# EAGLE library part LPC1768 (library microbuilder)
LPC1768 100 MHz 32-bit ARM Cortex-M3 based microcontroller featuring a high level of integration and low power consumption. 512 kB Flash, 64 kB SRAM, USB Device/Host/OTG, Ethernet, CAN, I2S, 10-bit DAC Digikey: 568-4796-ND
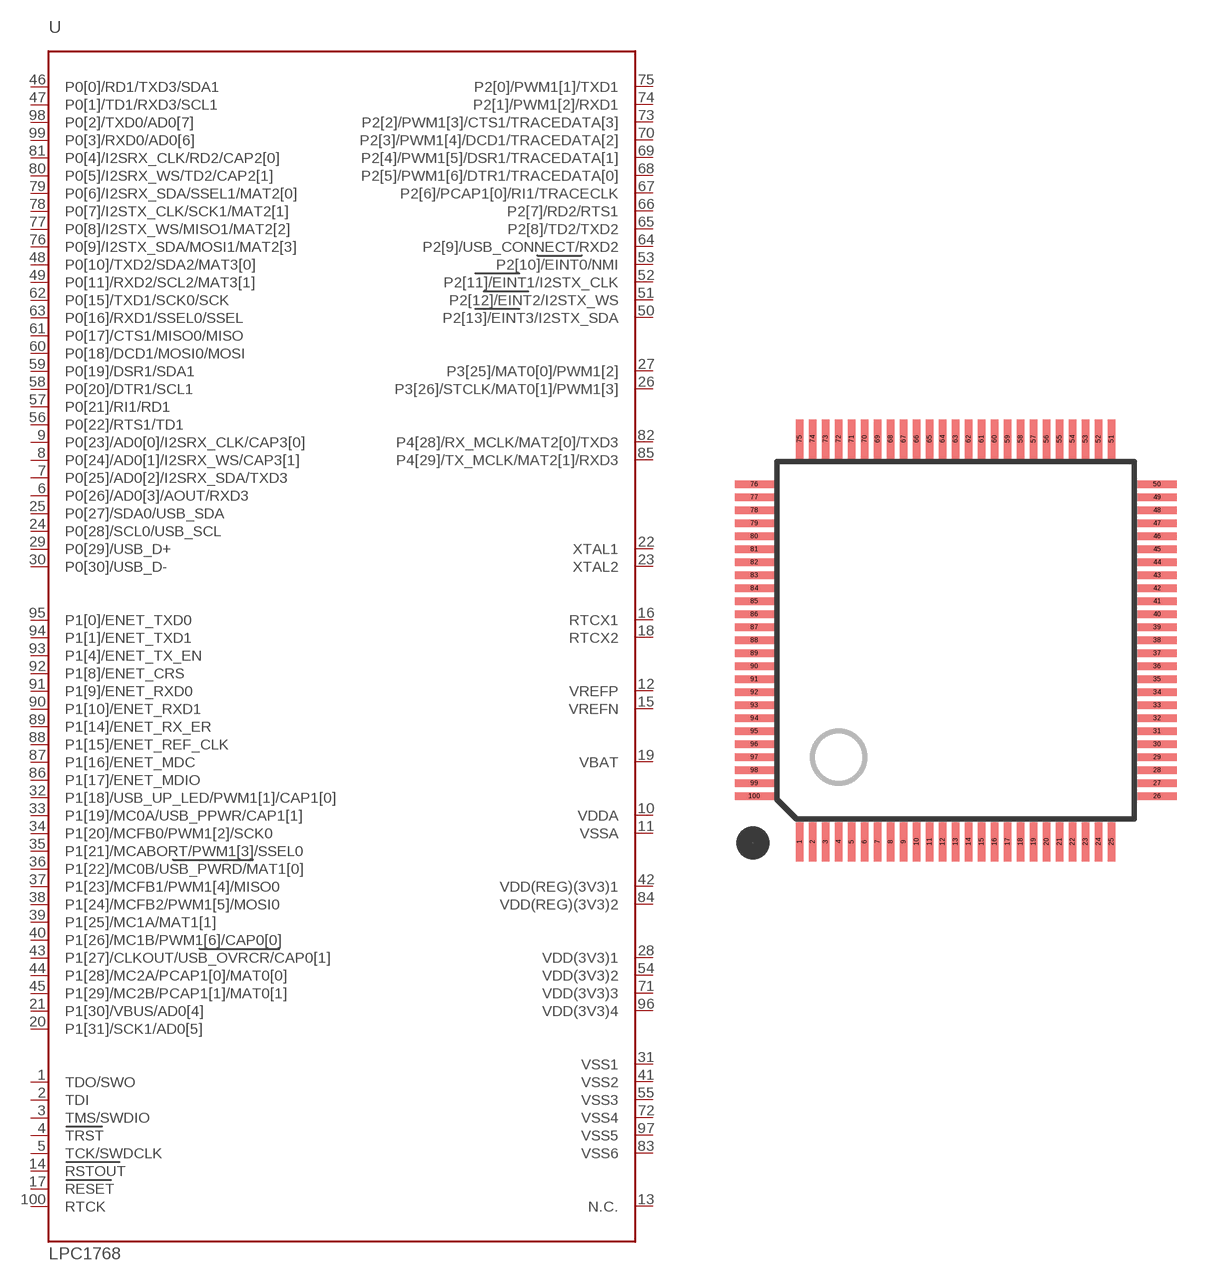
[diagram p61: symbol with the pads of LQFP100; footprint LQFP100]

Designator prefix U

## LPC1768  [LQFP100]
1  TDO/SWO
2  TDI
3  TMS/SWDIO
4  TRST
5  TCK/SWDCLK
6  P0[26]/AD0[3]/AOUT/RXD3
7  P0[25]/AD0[2]/I2SRX_SDA/TXD3
8  P0[24]/AD0[1]/I2SRX_WS/CAP3[1]
9  P0[23]/AD0[0]/I2SRX_CLK/CAP3[0]
10  VDDA  pwr
11  VSSA  pwr
12  VREFP  pwr
13  N.C.  nc
14  RSTOUT
15  VREFN  pwr
16  RTCX1
17  RESET
18  RTCX2
19  VBAT  pwr
20  P1[31]/SCK1/AD0[5]
21  P1[30]/VBUS/AD0[4]
22  XTAL1
23  XTAL2
24  P0[28]/SCL0/USB_SCL
25  P0[27]/SDA0/USB_SDA
26  P3[26]/STCLK/MAT0[1]/PWM1[3]
27  P3[25]/MAT0[0]/PWM1[2]
28  VDD(3V3)1  pwr
29  P0[29]/USB_D+
30  P0[30]/USB_D-
31  VSS1  pwr
32  P1[18]/USB_UP_LED/PWM1[1]/CAP1[0]
33  P1[19]/MC0A/USB_PPWR/CAP1[1]
34  P1[20]/MCFB0/PWM1[2]/SCK0
35  P1[21]/MCABORT/PWM1[3]/SSEL0
36  P1[22]/MC0B/USB_PWRD/MAT1[0]
37  P1[23]/MCFB1/PWM1[4]/MISO0
38  P1[24]/MCFB2/PWM1[5]/MOSI0
39  P1[25]/MC1A/MAT1[1]
40  P1[26]/MC1B/PWM1[6]/CAP0[0]
41  VSS2  pwr
42  VDD(REG)(3V3)1  pwr
43  P1[27]/CLKOUT/USB_OVRCR/CAP0[1]
44  P1[28]/MC2A/PCAP1[0]/MAT0[0]
45  P1[29]/MC2B/PCAP1[1]/MAT0[1]
46  P0[0]/RD1/TXD3/SDA1
47  P0[1]/TD1/RXD3/SCL1
48  P0[10]/TXD2/SDA2/MAT3[0]
49  P0[11]/RXD2/SCL2/MAT3[1]
50  P2[13]/EINT3/I2STX_SDA
51  P2[12]/EINT2/I2STX_WS
52  P2[11]/EINT1/I2STX_CLK
53  P2[10]/EINT0/NMI
54  VDD(3V3)2  pwr
55  VSS3  pwr
56  P0[22]/RTS1/TD1
57  P0[21]/RI1/RD1
58  P0[20]/DTR1/SCL1
59  P0[19]/DSR1/SDA1
60  P0[18]/DCD1/MOSI0/MOSI
61  P0[17]/CTS1/MISO0/MISO
62  P0[15]/TXD1/SCK0/SCK
63  P0[16]/RXD1/SSEL0/SSEL
64  P2[9]/USB_CONNECT/RXD2
65  P2[8]/TD2/TXD2
66  P2[7]/RD2/RTS1
67  P2[6]/PCAP1[0]/RI1/TRACECLK
68  P2[5]/PWM1[6]/DTR1/TRACEDATA[0]
69  P2[4]/PWM1[5]/DSR1/TRACEDATA[1]
70  P2[3]/PWM1[4]/DCD1/TRACEDATA[2]
71  VDD(3V3)3  pwr
72  VSS4  pwr
73  P2[2]/PWM1[3]/CTS1/TRACEDATA[3]
74  P2[1]/PWM1[2]/RXD1
75  P2[0]/PWM1[1]/TXD1
76  P0[9]/I2STX_SDA/MOSI1/MAT2[3]
77  P0[8]/I2STX_WS/MISO1/MAT2[2]
78  P0[7]/I2STX_CLK/SCK1/MAT2[1]
79  P0[6]/I2SRX_SDA/SSEL1/MAT2[0]
80  P0[5]/I2SRX_WS/TD2/CAP2[1]
81  P0[4]/I2SRX_CLK/RD2/CAP2[0]
82  P4[28]/RX_MCLK/MAT2[0]/TXD3
83  VSS6  pwr
84  VDD(REG)(3V3)2  pwr
85  P4[29]/TX_MCLK/MAT2[1]/RXD3
86  P1[17]/ENET_MDIO
87  P1[16]/ENET_MDC
88  P1[15]/ENET_REF_CLK
89  P1[14]/ENET_RX_ER
90  P1[10]/ENET_RXD1
91  P1[9]/ENET_RXD0
92  P1[8]/ENET_CRS
93  P1[4]/ENET_TX_EN
94  P1[1]/ENET_TXD1
95  P1[0]/ENET_TXD0
96  VDD(3V3)4  pwr
97  VSS5  pwr
98  P0[2]/TXD0/AD0[7]
99  P0[3]/RXD0/AD0[6]
100  RTCK

## Footprint LQFP100 (pad centres in mm)
LQFP100 Low Profile Quad Flat Package 14x14x1.4 mm
smd 0.27 x 1.5: 1 -6,-7.75; 2 -5.5,-7.75; 3 -5,-7.75; 4 -4.5,-7.75; 5 -4,-7.75; 6 -3.5,-7.75; 7 -3,-7.75; 8 -2.5,-7.75; 9 -2,-7.75; 10 -1.5,-7.75; 11 -1,-7.75; 12 -0.5,-7.75; 13 0,-7.75; 14 0.5,-7.75; 15 1,-7.75; 16 1.5,-7.75; 17 2,-7.75; 18 2.5,-7.75; 19 3,-7.75; 20 3.5,-7.75; 21 4,-7.75; 22 4.5,-7.75; 23 5,-7.75; 24 5.5,-7.75; 25 6,-7.75; 51 6,7.75; 52 5.5,7.75; 53 5,7.75; 54 4.5,7.75; 55 4,7.75; 56 3.5,7.75; 57 3,7.75; 58 2.5,7.75; 59 2,7.75; 60 1.5,7.75; 61 1,7.75; 62 0.5,7.75; 63 0,7.75; 64 -0.5,7.75; 65 -1,7.75; 66 -1.5,7.75; 67 -2,7.75; 68 -2.5,7.75; 69 -3,7.75; 70 -3.5,7.75; 71 -4,7.75; 72 -4.5,7.75; 73 -5,7.75; 74 -5.5,7.75; 75 -6,7.75
smd 1.5 x 0.27: 26 7.75,-6; 27 7.75,-5.5; 28 7.75,-5; 29 7.75,-4.5; 30 7.75,-4; 31 7.75,-3.5; 32 7.75,-3; 33 7.75,-2.5; 34 7.75,-2; 35 7.75,-1.5; 36 7.75,-1; 37 7.75,-0.5; 38 7.75,0; 39 7.75,0.5; 40 7.75,1; 41 7.75,1.5; 42 7.75,2; 43 7.75,2.5; 44 7.75,3; 45 7.75,3.5; 46 7.75,4; 47 7.75,4.5; 48 7.75,5; 49 7.75,5.5; 50 7.75,6; 76 -7.75,6; 77 -7.75,5.5; 78 -7.75,5; 79 -7.75,4.5; 80 -7.75,4; 81 -7.75,3.5; 82 -7.75,3; 83 -7.75,2.5; 84 -7.75,2; 85 -7.75,1.5; 86 -7.75,1; 87 -7.75,0.5; 88 -7.75,0; 89 -7.75,-0.5; 90 -7.75,-1; 91 -7.75,-1.5; 92 -7.75,-2; 93 -7.75,-2.5; 94 -7.75,-3; 95 -7.75,-3.5; 96 -7.75,-4; 97 -7.75,-4.5; 98 -7.75,-5; 99 -7.75,-5.5; 100 -7.75,-6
